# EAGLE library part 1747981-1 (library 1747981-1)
HDMI Receptacle Connector 19 Position Panel Mount; Surface Mount, Right Angle; Through Hole Source: Datasheet
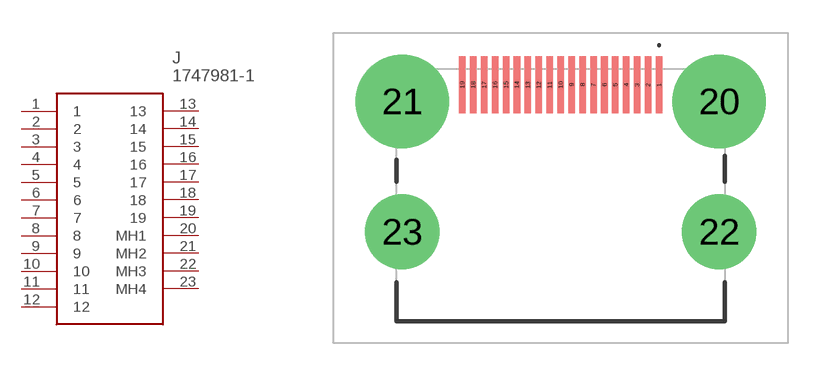
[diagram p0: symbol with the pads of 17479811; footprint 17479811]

Designator prefix J

## 1747981-1 (Description: HDMI Receptacle Connector 19 Position Panel Mount; Surface Mount, Right Angle; Through Hole; Height: 6.38mm; Manufacturer_Name: TE Connectivity; Manufacturer_Part_Number: 1747981-1)  [17479811]
1  1
2  2
3  3
4  4
5  5
6  6
7  7
8  8
9  9
10  10
11  11
12  12
13  13
14  14
15  15
16  16
17  17
18  18
19  19
20  MH1
21  MH2
22  MH3
23  MH4

## Footprint 17479811 (pad centres in mm)
1747981-1-4
smd 0.3 x 2.6: 1 4.5,5.035; 2 4,5.035; 3 3.5,5.035; 4 3,5.035; 5 2.5,5.035; 6 2,5.035; 7 1.5,5.035; 8 1,5.035; 9 0.5,5.035; 10 0,5.035; 11 -0.5,5.035; 12 -1,5.035; 13 -1.5,5.035; 14 -2,5.035; 15 -2.5,5.035; 16 -3,5.035; 17 -3.5,5.035; 18 -4,5.035; 19 -4.5,5.035
drill 2.85 pad 4.275: 20 7.25,4.275; 21 -7.25,4.275
drill 2.28 pad 3.42: 22 7.25,-1.685; 23 -7.25,-1.685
